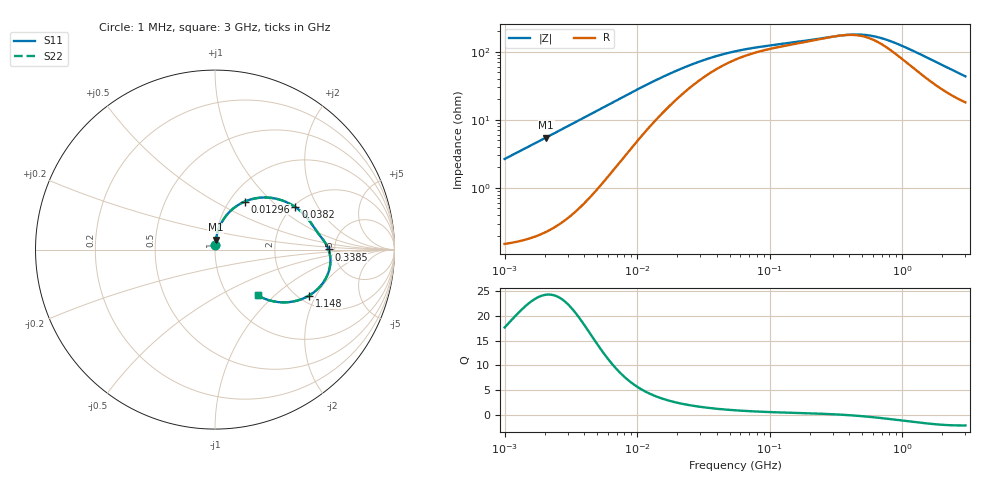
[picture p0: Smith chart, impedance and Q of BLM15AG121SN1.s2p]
! BLM15AG121SN1
# Hz S RI R 50
!Freq.(Hz) S11(Real) S11(Imag) S21(Real) S21(Imag) S12(Real) S12(Imag) S22(Real) S22(Imag)
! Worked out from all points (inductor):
!   401 points, 1 MHz to 3 GHz, reference 50 ohm
!   read as one part in series: L = 423 nH near 1.041 MHz
!   highest Q = 24.3 at 2.056 MHz (marker M1), where L = 424 nH
!   self-resonance near 340.6 MHz
!   S11 on the Smith chart (normalised r, x): 1 MHz: 1.00, +0.05; 12.96 MHz: 1.17, +0.70; 38.2 MHz: 2.06, +1.31; 338.5 MHz: 4.44, +0.01; 1.148 GHz: 2.26, -1.75; 3 GHz: 1.36, -0.79
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1000000  0.0022 0.0264  0.9978 -0.0264  0.9978 -0.0264  0.0022 0.0264
2055611  0.00523 0.0544  0.9948 -0.0544  0.9948 -0.0544  0.00523 0.0544
3823119  0.0158 0.1011  0.9842 -0.1011  0.9842 -0.1011  0.0158 0.1011
7400828  0.0604 0.1867  0.9396 -0.1867  0.9396 -0.1867  0.0604 0.1867
9794439  0.1032 0.2301  0.8968 -0.2301  0.8968 -0.2301  0.1032 0.2301
1.29622e7  0.1652 0.2674  0.8348 -0.2674  0.8348 -0.2674  0.1652 0.2674
1.461624e7  0.1968 0.2788  0.8032 -0.2788  0.8032 -0.2788  0.1968 0.2788
2.270269e7  0.3231 0.2868  0.6769 -0.2868  0.6769 -0.2868  0.3231 0.2868
3.820236e7  0.4479 0.2365  0.5521 -0.2365  0.5521 -0.2365  0.4479 0.2365
5.477226e7  0.5031 0.1881  0.4969 -0.1881  0.4969 -0.1881  0.5031 0.1881
9.593103e7  0.5522 0.1233  0.4478 -0.1233  0.4478 -0.1233  0.5522 0.1233
2.094008e8  0.6005 0.0574  0.3995 -0.0574  0.3995 -0.0574  0.6005 0.0574
3.385367e8  0.6324 0.000959  0.3676 -0.000959  0.3676 -0.000959  0.6324 0.000959
4.304467e8  0.6421 -0.0408  0.3579 0.0408  0.3579 0.0408  0.6421 -0.0408
5.258324e8  0.642 -0.0828  0.358 0.0828  0.358 0.0828  0.642 -0.0828
6.423554e8  0.6311 -0.1294  0.3689 0.1294  0.3689 0.1294  0.6311 -0.1294
8.005644e8  0.604 -0.1821  0.396 0.1821  0.396 0.1821  0.604 -0.1821
1.147801e9  0.5238 -0.2561  0.4762 0.2561  0.4762 0.2561  0.5238 -0.2561
1.430499e9  0.4577 -0.2841  0.5423 0.2841  0.5423 0.2841  0.4577 -0.2841
1.782824e9  0.3863 -0.2941  0.6137 0.2941  0.6137 0.2941  0.3863 -0.2941
2.221924e9  0.3174 -0.2864  0.6826 0.2864  0.6826 0.2864  0.3174 -0.2864
3e9  0.238 -0.2548  0.762 0.2548  0.762 0.2548  0.238 -0.2548
